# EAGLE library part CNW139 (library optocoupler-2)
HEWLETT PACKARD OPTO COUPLER
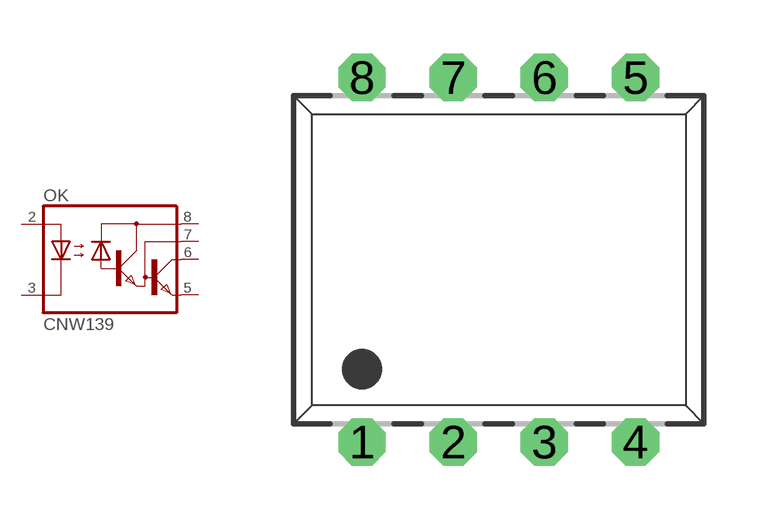
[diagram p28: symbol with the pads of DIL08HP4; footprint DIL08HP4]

Designator prefix OK

## CNW139  [DIL08HP4]
2  A  pas
3  C  pas
5  GND  pas
6  VO  pas
7  VB  pas
8  VCC  pas

## Footprint DIL08HP4 (pad centres in mm)
Dual In Line
drill 0.813 octagon: 1 -3.81,-5.08; 2 -1.27,-5.08; 3 1.27,-5.08; 4 3.81,-5.08; 5 3.81,5.08; 6 1.27,5.08; 7 -1.27,5.08; 8 -3.81,5.08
